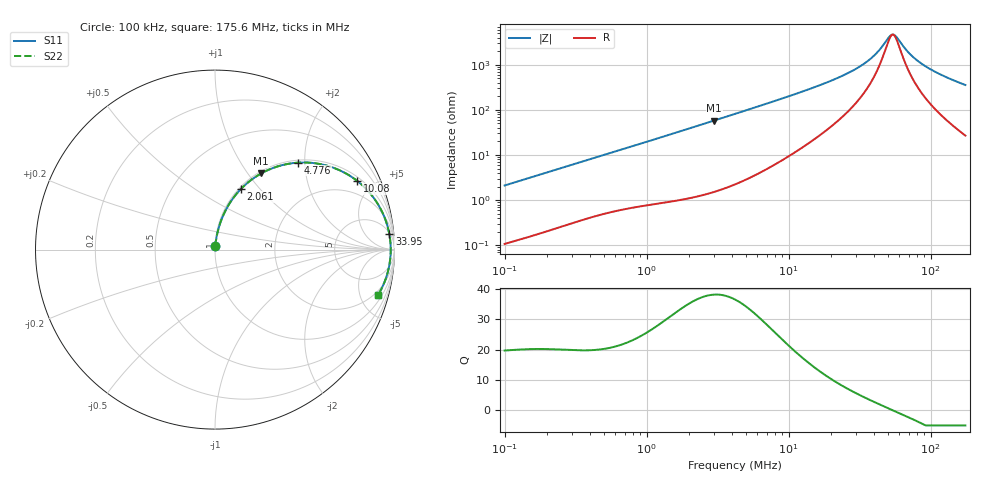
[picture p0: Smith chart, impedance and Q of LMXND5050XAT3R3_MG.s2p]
! LMXND5050XAT3R3_MG  S-PARAMETER MODEL  ( General Type )
! Model Generated by TAIYO YUDEN Corporation (http://www.ty-top.com)
! Version 1.0
! TAIYO YUDEN Control No. 191023NI43SB-FBB
! Copyright(c) 2019 TAIYO YUDEN CO.,LTD. All Rights Reserved.
! Product Description (link to TY-COMPAS)
! https://ds.yuden.co.jp/TYCOMPAS/or/detail?pn=LMXND5050XAT3R3MMG&u=M
! Products Name : Inductors
! Characteristics :
!  Inductance : 3.3 uH , SRF(min) : 36 MHz , DC Resistance(max) : 0.039 Ohm
!  Rated Current : Saturation :3600 mA , Temp Rise : 3000 mA
!  Case Size : 4.9 x 4.9 / 0.193 x 0.193 [mm/inch] , Thickness : 3.1 / 0.122 [mm/inch]
!  (Conditions: Temperature = 25 degC , DC Bias Current/Voltage = 0A / 0V)
! External Node Assignments :
!  1  o---GGG---o  2
! GND o---------o GND
! Frequency Range : 0.1MHz  -  175.64884MHz  [ 402 STEP ]
# MHz S RI R 50
! Freq[MHz].  S11 Real  S11 Imag  S21 Real  S21 Imag  S12 Real  S12 Imag  S22 Real  S22 Imag
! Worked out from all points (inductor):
!   401 points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, 100 kHz to 175.6 MHz, reference 50 ohm
!   read as one part in series: L = 3.34 uH near 103.8 kHz
!   highest Q = 38.1 at 2.994 MHz (marker M1), where L = 3.09 uH
!   self-resonance near 54.16 MHz
!   S11 on the Smith chart (normalised r, x): 100 kHz: 1.00, +0.04; 2.061 MHz: 1.02, +0.80; 4.776 MHz: 1.05, +1.86; 10.08 MHz: 1.19, +4.03; 33.95 MHz: 6, +20; 175.6 MHz: 1.54, -7.09
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0.1  0.00152 0.0211  0.9985 -0.0211  0.9985 -0.0211  0.00152 0.0211
0.349525  0.00855 0.0702  0.9914 -0.0702  0.9914 -0.0702  0.00855 0.0702
0.684693  0.0239 0.1316  0.9761 -0.1316  0.9761 -0.1316  0.0239 0.1316
1.221676  0.0609 0.2221  0.9391 -0.2221  0.9391 -0.2221  0.0609 0.2221
2.061016  0.1449 0.3383  0.8551 -0.3383  0.8551 -0.3383  0.1449 0.3383
2.994426  0.258 0.4246  0.742 -0.4246  0.742 -0.4246  0.258 0.4246
4.270063  0.4105 0.4783  0.5895 -0.4783  0.5895 -0.4783  0.4105 0.4783
4.776436  0.4648 0.4846  0.5352 -0.4846  0.5352 -0.4846  0.4648 0.4846
6.685178  0.6279 0.4665  0.3721 -0.4665  0.3721 -0.4665  0.6279 0.4665
10.0825  0.7914 0.3833  0.2086 -0.3833  0.2086 -0.3833  0.7914 0.3833
14.64875  0.8871 0.2843  0.1129 -0.2843  0.1129 -0.2843  0.8871 0.2843
23.80689  0.9508 0.1633  0.0492 -0.1633  0.0492 -0.1633  0.9508 0.1633
33.94871  0.971 0.088  0.029 -0.088  0.029 -0.088  0.971 0.088
41.69184  0.9767 0.0484  0.0233 -0.0484  0.0233 -0.0484  0.9767 0.0484
51.20104  0.979 0.0103  0.021 -0.0103  0.021 -0.0103  0.979 0.0103
54.15189  0.9791 1.49e-05  0.0209 -1.49e-05  0.0209 -1.49e-05  0.9791 1.49e-05
56.21301  0.9791 -0.00683  0.0209 0.00683  0.0209 0.00683  0.9791 -0.00683
71.66182  0.9764 -0.0519  0.0236 0.0519  0.0236 0.0519  0.9764 -0.0519
80.15997  0.9736 -0.0733  0.0264 0.0733  0.0264 0.0733  0.9736 -0.0733
93.07873  0.9682 -0.103  0.0318 0.103  0.0318 0.103  0.9682 -0.103
125.4978  0.9495 -0.1676  0.0505 0.1676  0.0505 0.1676  0.9495 -0.1676
175.6488  0.9104 -0.2502  0.0896 0.2502  0.0896 0.2502  0.9104 -0.2502
